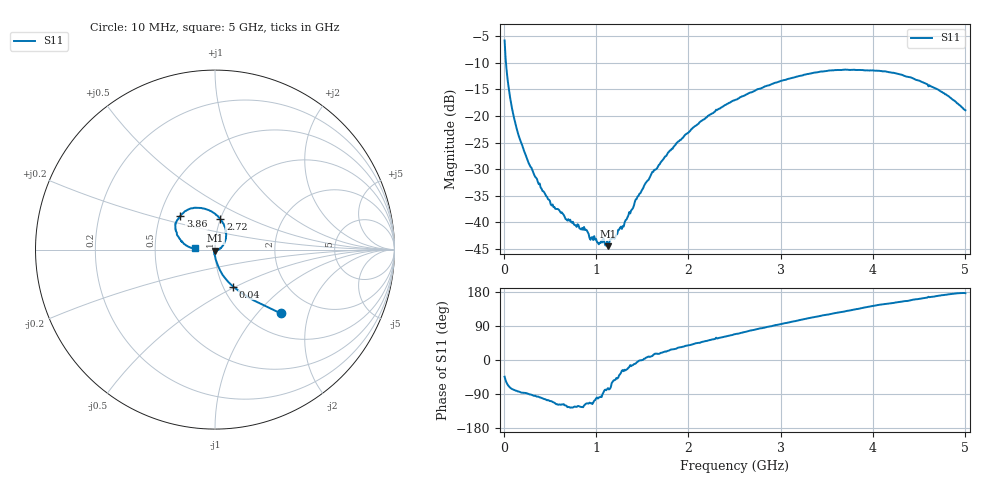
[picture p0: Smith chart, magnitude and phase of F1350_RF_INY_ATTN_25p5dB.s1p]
! S-parameters for RF_INY input IDT F1350 DPD Demodulator
! Date Measured:  2015-11-25  RGG
!  Port 1 = Pin 3 = RF_INY
! STATE: RF_INY selected, 25.5 dB attenuation (Gain = Gmax - 25.5 dB)
! RF Frequency:  10 MHz to 5000 MHz
! RF_INX, IF_I+, IF_I-, IF_Q+, and IF_Q- terminated
! 2300 MHz, 0 dBm signal applied to LO_IN
! Vcc = +5.00 Volts  Icc = approx 275 mA
! NOTES:  The device was measured on a custom printed circuit evaluation board with individual 50 ohm
!  microstrip lines to the RF and LO pins. The 50 ohm microstrip lines were de-embedded using reference
!  plane extensions
! Device Description:  F1350 RF_INX ATTN=0dB RF_INX selected
! Instrument Manufacturer:  Agilent Technologies
! Instrument Model:  E5071C
! Instrument Serial Number:  MY46419053
! Instrument Firmware Rev:  A.11.31
# HZ  S  RI R 50.00
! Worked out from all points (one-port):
!   500 points, 10 MHz to 5 GHz, reference 50 ohm
!   lowest |S11| = -44.4 dB at 1.13 GHz (marker M1), VSWR 1.01, Z = 50.2 - j0.579 ohm
!   |S11| at or under -10 dB: 24.65 MHz to end of sweep
!   S11 on the Smith chart (normalised r, x): 10 MHz: 1.40, -1.34; 40 MHz: 1.11, -0.49; 2.72 GHz: 1.00, +0.35; 3.86 GHz: 0.64, +0.26; 5 GHz: 0.80, +0.01
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1e7  0.3659 -0.3552
4e7  0.1013 -0.2063
7e7  0.0426 -0.1415
1.2e8  0.0157 -0.0882
1.7e8  0.00676 -0.0619
2.6e8  0.00087 -0.038
4e8  -0.00337 -0.021
5e8  -0.005 -0.0152
6.4e8  -0.00554 -0.0107
6.9e8  -0.00588 -0.00859
8.9e8  -0.00369 -0.00773
9.5e8  -0.0029 -0.00662
1.13e9  0.00163 -0.00577
1.26e9  0.00708 -0.00544
1.3e9  0.00797 -0.00453
1.44e9  0.0165 -0.00184
1.61e9  0.0293 0.00544
1.89e9  0.0484 0.0311
2.23e9  0.0622 0.0814
2.51e9  0.0523 0.1315
2.72e9  0.0301 0.1696
3.13e9  -0.0457 0.2234
3.43e9  -0.1155 0.2326
3.76e9  -0.1783 0.2029
3.86e9  -0.1938 0.1872
4.38e9  -0.2124 0.0941
4.7e9  -0.1741 0.0327
5e9  -0.1126 0.00717
